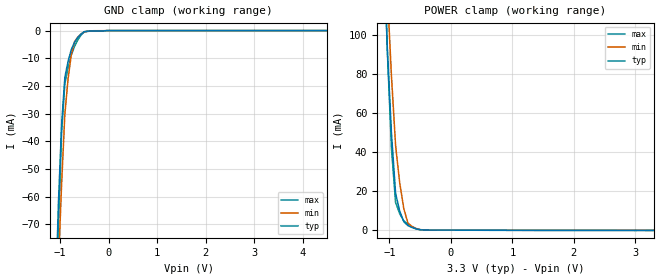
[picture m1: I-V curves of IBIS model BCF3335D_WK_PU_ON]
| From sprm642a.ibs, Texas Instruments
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|BCF3335D_WK_PD_ON; WEAK_PULLDOWN_ON
|   Model Cell BCF3335D_WK_PU_ON
|BCF3335D_WK_PU_ON
[Model]   BCF3335D_WK_PU_ON
Model_type   Input
Polarity   Non-Inverting
Vinl =  0.8
Vinh =  2
C_comp   1.199917p   1.06526p   1.338254p
[Model Spec]
Vinl   0.8   0.8   0.8
Vinh   2   2   2
[Temperature Range]   25   155   -40
[Voltage Range]   3.3   2.97   3.63
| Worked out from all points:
|   GND clamp passes 1 mA (typ) near -0.55 V on its own axis
|   POWER clamp passes 1 mA (typ) near -0.60 V on its own axis
| Nom Voltages:
|   VDD=1.2, VDDS=3.3, VSS=0
| Min Voltages:
|   VDD=1.08, VDDS=2.97, VSS=0
| Max Voltages:
|   VDD=1.32, VDDS=3.63, VSS=0
[POWER_clamp]
|   voltage   I(typ)   I(min)   I(max)
-3.3V     2.333A     2.602A     3.083A
-1.1V     147.5mA    172.2mA    162.2mA
-1.033V   92.35mA    121.7mA    91.22mA
-966.7mV  49.49mA    78.85mA    41.87mA
-900mV    18.88mA    43.5mA     14.19mA
-833.3mV  9.819mA    24.38mA    8.478mA
-766.7mV  4.303mA    11.09mA    4.779mA
-700mV    2.33mA     3.648mA    3.088mA
-566.7mV  645.5uA    749.7uA    840.9uA
-500mV    187.9uA    260.4uA    219.6uA
-366.7mV  40.03uA    41.85uA    52.54uA
3.3V      -108.8uA   -62.59uA   -174uA
[GND_clamp]
|   voltage   I(typ)   I(min)   I(max)
-3.3V     -1.904A    -1.594A    -3.188A
-1.1V     -103.1mA   -119.1mA   -124mA
-1.033V   -62.9mA    -85.19mA   -71.77mA
-966.7mV  -34.17mA   -55.6mA    -36.9mA
-900mV    -16.95mA   -30.33mA   -19.33mA
-833.3mV  -11.11mA   -17.42mA   -13.36mA
-766.7mV  -6.867mA   -8.655mA   -8.824mA
-700mV    -4.21mA    -4.028mA   -5.714mA
-566.7mV  -1.238mA   -1.201mA   -1.653mA
-500mV    -399.1uA   -475uA     -506.7uA
-33.33mV  0A         0A         0A
6.6V      0A         0A         0A
